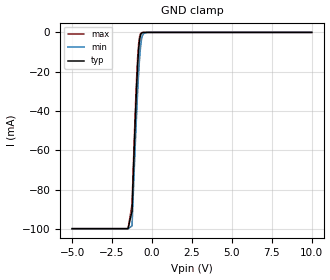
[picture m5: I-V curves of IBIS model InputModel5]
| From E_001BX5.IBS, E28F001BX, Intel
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|************************Input Model 5*************************************
[Model]   InputModel5
Model_type   Input
|   Model for pin A[11]
Vinl = 0.8V
Vinh = 2.0V
|Variable   Typ   Min   Max
C_comp   9.13p   7.20p   11.06p
[Voltage Range]   5.0V   4.5V   5.5V
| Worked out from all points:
|   GND clamp passes 1 mA (typ) near -0.70 V on its own axis
[GND_clamp]
|Voltage   I(typ)   I(min)   I(max)
-5V       -99.85mA   -99.85mA   -99.85mA
-1.5V     -99.85mA   -99.85mA   -99.85mA
-1.25V    -90.92mA   -98.47mA   -87.46mA
-1.05V    -45.04mA   -57.66mA   -40.38mA
-950mV    -25.16mA   -38.89mA   -20.53mA
-900mV    -16.84mA   -30.32mA   -12.61mA
-850mV    -10.24mA   -22.64mA   -6.798mA
-800mV    -5.363mA   -15.77mA   -3.052mA
-700mV    -998.4uA   -6.01mA    -410.7uA
-600mV    -121.1uA   -1.645mA   -44.5uA
-250mV    0A         0A         0A
10V       0A         0A         0A
[Power_clamp]
| Input buffer circuits of this product do not intrinisically
| require a [Power_clamp] defintion.  This zero current
| [Power_clamp] table is provided for compatibility with
| some IBIS parsers.
|Voltage   I(typ)   I(min)   I(max)
-5V       0A         0A         0A
0V        0A         0A         0A
5V        0A         0A         0A
10V       0A         0A         0A
